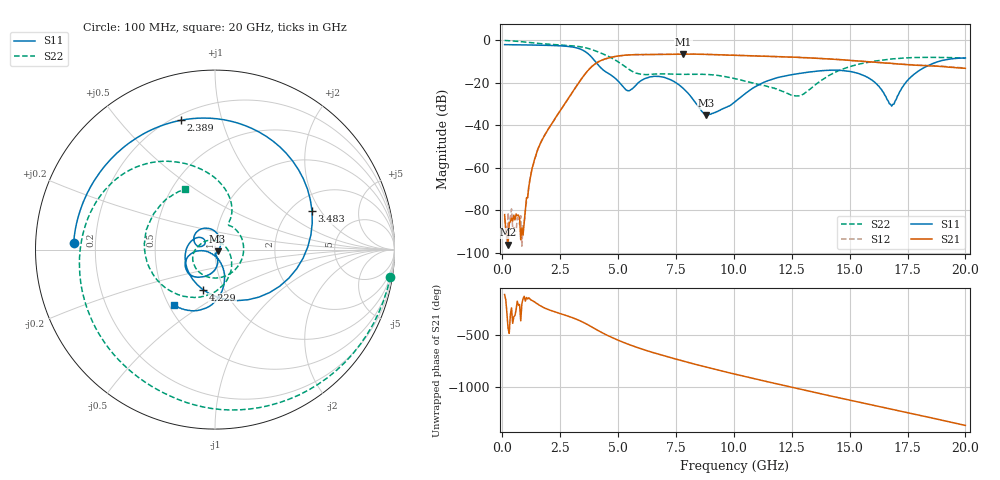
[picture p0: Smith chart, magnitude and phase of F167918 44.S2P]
!  2-Port S-parameters saved by WinCal
! VAR MeasName=S-Parameters (CALIBRATED_DATA) read from VNA (N5242A)
! VAR MeasDate=2016-11-22 10:26:55
! VAR NAME=F167918 44
! VAR FILENAME=F167918 44.S2P
! VAR DATE=2016-11-22 10:26:55
! VAR PHYS_PORTS=1,2
# Hz S DB R 50
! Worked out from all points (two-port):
!   401 points, 100 MHz to 20 GHz, reference 50 ohm
!   highest |S21| = -6.48 dB at 7.811 GHz (marker M1); lowest = -96.1 dB at 249.2 MHz (marker M2)
!   |S21| within 3 dB of the highest: 4.276 GHz to 15.06 GHz (10.78 GHz wide, 112 % of centre)
!   lowest |S11| = -35.2 dB at 8.806 GHz (marker M3), VSWR 1.04, Z = 51.4 - j1.02 ohm
!   |S11| at or under -10 dB: 4.018 GHz to 18.84 GHz (14.82 GHz wide, 130 % of centre)
!   |S22| runs from -26.2 to -0.1 dB; largest |S21 - S12| = 0.0061
!   S11 on the Smith chart (normalised r, x): 100 MHz: 0.12, +0.02; 2.389 GHz: 0.23, +0.74; 3.483 GHz: 2.58, +1.67; 4.229 GHz: 0.80, -0.37; 20 GHz: 0.53, -0.39
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1e8  -2.07 177.3  -82.01 -117.3  -83.76 -107.5  -0.10 -8.8
2.4925e8  -2.08 173.3  -96.13 -81.2  -81.14 117.1  -0.20 -21.0
9.4575e8  -2.19 154.6  -85.82 -134.1  -85.64 169.5  -0.78 -74.2
1.493e9  -2.29 138.5  -52.61 157.0  -52.57 156.0  -1.43 -109.5
2.3885e9  -2.56 104.8  -35.01 67.8  -35.01 67.8  -2.13 -157.0
3.43325e9  -4.45 27.6  -17.93 -16.6  -17.95 -16.5  -3.18 150.2
3.483e9  -4.71 21.6  -17.20 -21.9  -17.20 -21.8  -3.27 147.5
3.881e9  -8.24 -38.2  -12.25 -69.8  -12.21 -69.7  -4.43 126.1
4.22925e9  -12.66 -106.9  -9.71 -113.3  -9.67 -113.4  -5.89 109.2
5.12475e9  -20.72 137.2  -7.22 154.2  -7.24 154.0  -11.04 71.6
5.871e9  -19.99 168.4  -6.77 92.1  -6.76 92.0  -15.70 63.2
6.7665e9  -17.02 128.9  -6.65 30.4  -6.67 30.1  -15.86 37.4
7.81125e9  -22.61 70.6  -6.48 -34.5  -6.51 -34.5  -16.04 -37.0
8.80625e9  -35.21 -34.7  -6.65 -92.4  -6.66 -92.5  -16.04 -108.3
1.005e10  -28.92 -77.8  -7.04 -159.9  -7.05 -159.8  -18.08 -167.2
1.179125e10  -17.88 -96.1  -7.66 110.8  -7.63 110.8  -22.78 141.5
1.27365e10  -15.75 -112.6  -8.04 63.2  -8.01 63.2  -26.17 64.2
1.338325e10  -14.82 -122.3  -8.37 30.8  -8.31 30.8  -22.18 -8.0
1.557225e10  -16.37 -166.6  -9.88 -76.5  -9.93 -77.1  -10.85 -111.9
1.67165e10  -29.90 -147.5  -10.79 -131.9  -10.86 -131.6  -8.92 -148.3
1.815925e10  -13.21 -78.1  -11.88 160.1  -11.77 160.3  -8.05 169.2
2e10  -8.31 -126.2  -13.21 69.1  -13.08 68.6  -8.51 116.7
